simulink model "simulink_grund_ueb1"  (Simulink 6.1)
settings: Solver=ode45  StartTime=0.0  StopTime=10.0  RelTol=1e-3

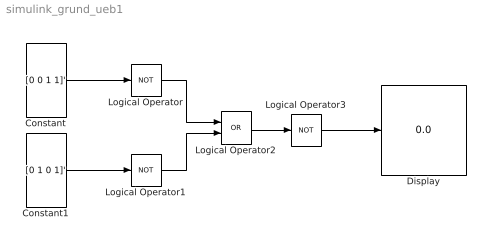
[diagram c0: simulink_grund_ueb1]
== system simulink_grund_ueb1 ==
  Constant : Constant  Value=[0 0 1 1]'  VectorParams1D=off  OutDataTypeMode=boolean
  Constant1 : Constant  Value=[0 1 0 1]'  VectorParams1D=off  OutDataTypeMode=boolean
  Display : Display
  Logical Operator : Logic  Operator=NOT  AllPortsSameDT=off  OutDataTypeMode=Boolean
  Logical Operator1 : Logic  Operator=NOT  AllPortsSameDT=off  OutDataTypeMode=Boolean
  Logical Operator2 : Logic  Operator=OR  AllPortsSameDT=off  OutDataTypeMode=Boolean
  Logical Operator3 : Logic  Operator=NOT  AllPortsSameDT=off  OutDataTypeMode=Boolean
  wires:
  Constant/1 -> Logical Operator/1
  Logical Operator/1 -> Logical Operator2/1
  Constant1/1 -> Logical Operator1/1
  Logical Operator1/1 -> Logical Operator2/2
  Logical Operator2/1 -> Logical Operator3/1
  Logical Operator3/1 -> Display/1
